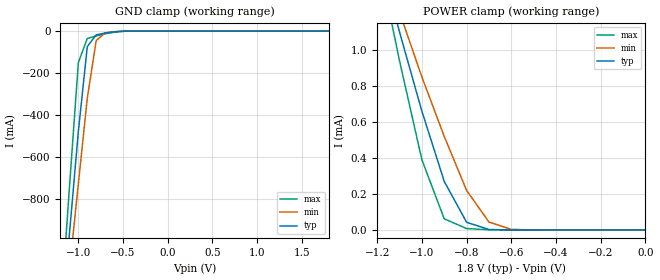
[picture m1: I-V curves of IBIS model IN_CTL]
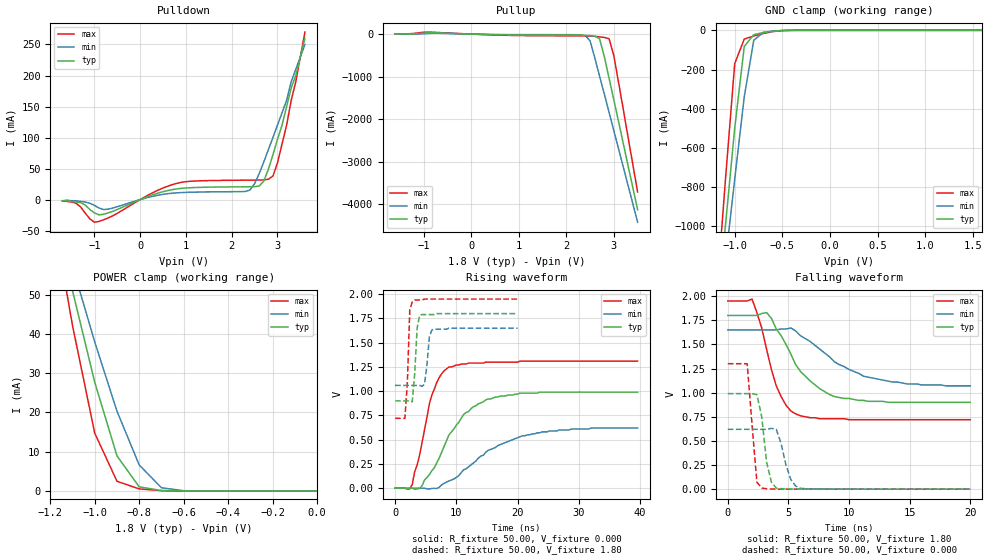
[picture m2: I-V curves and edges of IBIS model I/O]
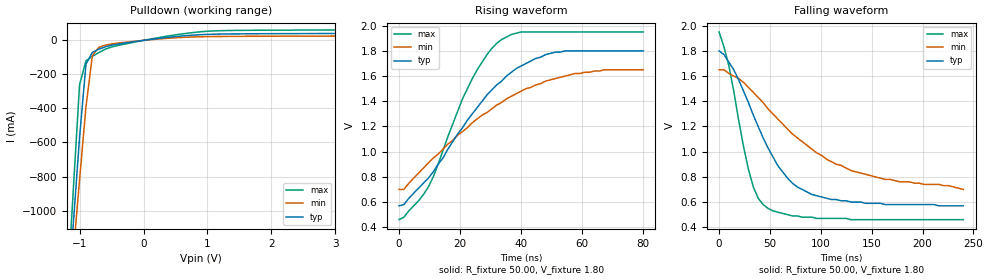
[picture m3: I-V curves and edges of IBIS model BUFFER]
| This IBIS file was created by s2ibis3 version 1.1
| North Carolina State University, ERL, 2006
[IBIS ver] 3.2
[File name] s34ms01g1_b_i_18_r2.ibs
[File Rev] 2.0
|   Rev1.0 Initial release with updated measurement
|   (X16 ONFI F48 98662AE 41087)
|   Rev2.0 Update 0A for 0V
[Date] 07/23/2014
[Source] Spansion IBIS team
|   Email: dl.ibisteam@spansion.com
[Notes]  Generated IBIS models from SPICE simulations.
|   VIO=1.65V - 1.95V, Temperature Range: Industrial (-40oC to +90oC).
[Disclaimer] THE MODEL LIBRARIES ARE PROVIDED AS IS.
[Copyright] (C) COPYRIGHT 2014
| SPANSION LLC
| ALL RIGHTS RESERVED.
|   Component S34MS01G1 X16 ONFI F48 in VBM063 package
[Component]   S34MS01G1
[Manufacturer]   Spansion
[Package]
| variable   typ   min   max
R_pkg   201.77mOhm   180.41mOhm   223.54mOhm
L_pkg   4.10nH   3.29nH   5.20nH
C_pkg   1.27pF   1.10pF   1.60pF
[Pin]   signal_name   model_name   R_pin   L_pin   C_pin
 A1   R   NC
 A2   R   NC
 A9   R   NC
 A10   R   NC
 B1   R   NC
 B9   R   NC
 B10   R   NC
 C3   WP#   BUFFER   223.54m   4.84n   1.60p
 C4   AL   IN_CTL   217.83m   4.92n   1.44p
 C5   VSS   GND
 C6   E#   IN_CTL   189.69m   3.65n   1.15p
 C7   W#   IN_CTL   210.13m   4.21n   1.36p
 C8   RB#   IN_CTL   180.41m   3.32n   1.18p
 D3   VDD   POWER
 D4   R#   IN_CTL   203.67m   4.50n   1.39p
 D5   CL   IN_CTL   192.84m   3.97n   1.24p
 D6   R   NC
 D7   R   NC
 D8   R   NC
 E3   R   NC
 E4   R   NC
 E5   R   NC
 E6   R   NC
 E7   R   NC
 E8   R   NC
 F3   R   NC
 F4   R   NC
 F5   R   NC
 F6   R   NC
 F7   VSS   GND
 F8   R   NC
 G3   R   NC
 G4   VDD   POWER
 G5   R   NC
 G6   I/O13   I/O   191.74m   3.47n   1.12p
 G7   I/O15   I/O   195.49m   3.29n   1.17p
 G8   R   NC
 H3   I/O8   I/O   213.66m   5.20n   1.43p
 H4   I/O0   I/O   209.17m   4.18n   1.39p
 H5   I/O10   I/O   185.98m   4.00n   1.10p
 H6   I/O12   I/O   198.14m   3.38n   1.18p
 H7   I/O14   I/O   191.63m   3.38n   1.16p
 H8   VDD   POWER
 J3   I/O9   I/O   212.31m   5.12n   1.41p
 J4   I/O1   I/O   204.93m   4.77n   1.32p
 J5   I/O11   I/O   196.16m   3.66n   1.14p
 J6   VDD   POWER
 J7   I/O5   I/O   195.51m   3.75n   1.19p
 J8   I/O7   I/O   199.84m   3.81n   1.17p
 K3   VSS   GND
 K4   I/O2   I/O   212.59m   4.62n   1.32p
 K5   I/O3   I/O   198.07m   3.97n   1.15p
 K6   I/O4   I/O   208.64m   4.08n   1.33p
 K7   I/O6   I/O   208.81m   4.22n   1.32p
 K8   VSS   GND
 L1   R   NC
 L2   R   NC
 L9   R   NC
 L10   R   NC
 M1   R   NC
 M2   R   NC
 M9   R   NC
 M10   R   NC
| Models and submodels in the file (3): IN_CTL (Input), I/O (I/O), BUFFER (Open_drain)
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|   Model IN_CTL
[Model]   IN_CTL
Model_type   Input
Vinl =   0.36V
Vinh =   1.44V
C_comp   4.34pF   3.91pF   5.21pF
[Temperature Range]   25.00   90.00   -40.00
[Voltage Range]   1.80V   1.65V   1.95V
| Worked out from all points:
|   GND clamp passes 1 mA (typ) near -0.50 V on its own axis
|   POWER clamp passes 1 mA (typ) near -1.08 V on its own axis
[GND_clamp]
| voltage   I(typ)   I(min)   I(max)
-1.8V     -4.43A     -4.03A     -5.05A
-1.2V     -1.47A     -1.56A     -1.36A
-1.1V     -970mA     -1.14A     -750mA
-1V       -480mA     -730mA     -150mA
-900mV    -73.87mA   -320mA     -35.7mA
-800mV    -17.88mA   -45.12mA   -23.11mA
-700mV    -9.1mA     -8.55mA    -13.23mA
-600mV    -3.69mA    -2.85mA    -5.42mA
-400mV    -110uA     -120uA     -100uA
1.8V      240pA      1.3nA      110pA
[POWER_clamp]
| voltage   I(typ)   I(min)   I(max)
-1.8V     4.52mA     3.92mA     5.46mA
-1.2V     1.57mA     1.59mA     1.54mA
-1.1V     1.1mA      1.21mA     940uA
-1V       660uA      850uA      390uA
-900mV    270uA      520uA      62.17uA
-800mV    42.85uA    220uA      7.81uA
-700mV    2.54uA     43.98uA    890nA
-600mV    180nA      3.36uA     66.87nA
0V        0A         0A         0A
|   Model I/O
[Model]   I/O
Model_type   I/O
Polarity   Inverting
Enable   Active-Low
Vinl  =   0.36V
Vinh  =   1.44V
Vmeas =   0.90V
C_comp   3.48pF   3.13pF   4.18pF
[Temperature Range]   25.00   90.00   -40.00
[Voltage Range]   1.80V   1.65V   1.95V
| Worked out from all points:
|   slope of the pulldown table from 0 to 0.27 V, typ, clamps not added: 35.9 ohm
|   slope of the pullup table from 0 to 0.27 V, typ, clamps not added: 31.6 ohm
|   GND clamp passes 1 mA (typ) near -0.49 V on its own axis
|   POWER clamp passes 1 mA (typ) near -0.80 V on its own axis
|   rising waveform, R_fixture 50.00, V_fixture 0.000: 20-80 % time 5.79ns typ, 8.76ns min, 2.87ns max; typ from 0 V to 0.99 V
|   rising waveform, R_fixture 50.00, V_fixture 1.80: 20-80 % time 512ps typ, 545ps min, 455ps max; typ from 0.9 V to 1.8 V
|   falling waveform, R_fixture 50.00, V_fixture 1.80: 20-80 % time 2.97ns typ, 4.24ns min, 1.66ns max; typ from 1.8 V to 0.9 V
|   falling waveform, R_fixture 50.00, V_fixture 0.000: 20-80 % time 630ps typ, 805ps min, 510ps max; typ from 0.99 V to 0 V
[Pulldown]
| voltage   I(typ)   I(min)   I(max)
-1.7V     -2mA       -2mA       -2mA
-1.4V     -4mA       -2mA       -6mA
-1V       -21.5mA    -9.4mA     -36.5mA
-700mV    -21.55mA   -15.49mA   -29.61mA
800mV     17.17mA    10.84mA    26.12mA
2.3V      20.58mA    13.03mA    31.25mA
2.5V      20.78mA    25.63mA    31.37mA
2.7V      29.72mA    60.45mA    31.69mA
2.9V      71.92mA    100mA      37.76mA
3.2V      150mA      160mA      120mA
3.3V      180mA      190mA      160mA
3.6V      260mA      250mA      270mA
[Pullup]
| voltage   I(typ)   I(min)   I(max)
-1.6V     2.6mA      1.9mA      3.3mA
-900mV    30.55mA    14.19mA    46.85mA
700mV     -18.21mA   -11.31mA   -27.49mA
2.1V      -24.45mA   -14.19mA   -41.16mA
2.4V      -29.59mA   -34.69mA   -42.55mA
2.5V      -36.59mA   -160mA     -45.69mA
2.6V      -47.63mA   -560mA     -53.7mA
2.7V      -110mA     -990mA     -65.37mA
2.8V      -530mA     -1.41A     -79.35mA
2.9V      -1.04A     -1.84A     -110mA
3V        -1.55A     -2.27A     -510mA
3.5V      -4.13A     -4.42A     -3.71A
[GND_clamp]
| voltage   I(typ)   I(min)   I(max)
-1.6V     -3.59A     -3.33A     -3.99A
-1.2V     -1.52A     -1.61A     -1.42A
-1.1V     -1.01A     -1.19A     -780mA
-1V       -500mA     -760mA     -170mA
-900mV    -82.68mA   -340mA     -44.8mA
-800mV    -22.28mA   -50.64mA   -28.91mA
-700mV    -11.42mA   -10.58mA   -16.3mA
-600mV    -4.6mA     -3.62mA    -6.52mA
-400mV    -130uA     -150uA     -120uA
1.6V      290pA      1.71nA     140pA
[POWER_clamp]
| voltage   I(typ)   I(min)   I(max)
-1.8V     240mA      210mA      290mA
-1.2V     76.17mA    77.46mA    74.6mA
-1.1V     51.04mA    57.29mA    42.14mA
-1V       27.7mA     37.97mA    14.73mA
-900mV    8.94mA     20.33mA    2.46mA
-800mV    1.03mA     6.62mA     520uA
-700mV    97.74uA    810uA      68.2uA
-600mV    10.52uA    59.01uA    5.35uA
0V        0A         0A         0A
[Ramp]
| variable   typ   min   max
dV/dt_r   0.58/5.46n   0.31/6.36n   0.78/2.81n
dV/dt_f   0.54/2.91n   0.35/4.33n   0.74/1.55n
R_load = 50.00
[Rising Waveform]
R_fixture = 50.00
V_fixture = 0.000
V_fixture_min = 0.000
V_fixture_max = 0.000
| time   V(typ)   V(min)   V(max)
0s        0V         0V         0V
2.8ns     -26uV      220nV      37.73mV
4ns       -2.35mV    79.58uV    340mV
6ns       180mV      -2.61mV    960mV
7.2ns     310mV      8.53mV     1.14V
8.8ns     550mV      74.68mV    1.25V
11.2ns    760mV      190mV      1.28V
16.4ns    940mV      420mV      1.3V
24ns      990mV      580mV      1.31V
39.6ns    990mV      620mV      1.31V
[Rising Waveform]
R_fixture = 50.00
V_fixture = 1.80
V_fixture_min = 1.65
V_fixture_max = 1.95
| time   V(typ)   V(min)   V(max)
0s        900mV      1.06V      720mV
1.6ns     900mV      1.06V      720mV
2ns       900mV      1.06V      1.08V
2.4ns     900mV      1.06V      1.84V
2.8ns     890mV      1.06V      1.92V
3.6ns     1.65V      1.06V      1.94V
4ns       1.78V      1.06V      1.94V
4.8ns     1.79V      1.07V      1.95V
6ns       1.79V      1.63V      1.95V
20ns      1.8V       1.65V      1.95V
[Falling Waveform]
R_fixture = 50.00
V_fixture = 1.80
V_fixture_min = 1.65
V_fixture_max = 1.95
| time   V(typ)   V(min)   V(max)
0s        1.8V       1.65V      1.95V
2ns       1.8V       1.65V      1.97V
2.8ns     1.82V      1.65V      1.67V
3.2ns     1.83V      1.65V      1.45V
4ns       1.66V      1.65V      1.07V
4.8ns     1.5V       1.66V      870mV
5.6ns     1.29V      1.64V      780mV
8.4ns     980mV      1.37V      730mV
11.2ns    920mV      1.17V      720mV
20ns      900mV      1.07V      720mV
[Falling Waveform]
R_fixture = 50.00
V_fixture = 0.000
V_fixture_min = 0.000
V_fixture_max = 0.000
| time   V(typ)   V(min)   V(max)
0s        990mV      620mV      1.3V
1.6ns     990mV      620mV      1.3V
2.4ns     980mV      620mV      72.85mV
2.8ns     750mV      620mV      12.43mV
3.2ns     280mV      620mV      3.88mV
3.6ns     71.09mV    630mV      1.96mV
4ns       10.62mV    620mV      1.11mV
5.2ns     1.94mV     99.79mV    380uV
6ns       760uV      8.29mV     190uV
20ns      35.13uV    13.85uV    10.73uV
|   Model BUFFER
[Model]   BUFFER
Model_type   Open_drain
Polarity   Non-Inverting
Enable   Active-Low
Vmeas =   0.9000V
Rref =   2.0000k
Vref =   1.8000V
C_comp   3.92pF   3.53pF   4.70pF
[Temperature Range]   25.00   90.00   -40.00
[Voltage Range]   1.80V   1.65V   1.95V
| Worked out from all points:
|   slope of the pulldown table from 0 to 0.27 V, typ, clamps not added: 20.7 ohm
|   rising waveform, R_fixture 50.00, V_fixture 1.80: 20-80 % time 22.8ns typ, 29.6ns min, 15.3ns max; typ from 0.57 V to 1.8 V
|   falling waveform, R_fixture 50.00, V_fixture 1.80: 20-80 % time 44.7ns typ, 85.2ns min, 22ns max; typ from 1.8 V to 0.57 V
[Pulldown]
| voltage   I(typ)   I(min)   I(max)
-1.7V     -4.29A     -3.92A     -4.86A
-1.2V     -1.62A     -1.7A      -1.54A
-1.1V     -1.09A     -1.26A     -890mA
-1V       -570mA     -820mA     -260mA
-900mV    -140mA     -390mA     -120mA
-800mV    -70.59mA   -90.34mA   -94.24mA
-700mV    -51.91mA   -41.16mA   -71.52mA
-400mV    -21.65mA   -15.79mA   -29.77mA
300mV     14.37mA    9.95mA     20.49mA
900mV     33.57mA    21.29mA    50.74mA
1.5V      38.33mA    23.73mA    58.75mA
3.6V      40.97mA    25.68mA    61.9mA
[Ramp]
| variable   typ   min   max
dV/dt_r   0.36/11.11n   0.26/11.19n   0.55/9.56n
dV/dt_f   0.15/11.48n   50.40m/10.06n   0.44/11.38n
R_load = 50.00
[Rising Waveform]
R_fixture = 50.00
V_fixture = 1.80
V_fixture_min = 1.65
V_fixture_max = 1.95
| time   V(typ)   V(min)   V(max)
0s        570mV      700mV      460mV
1.6ns     580mV      700mV      480mV
9.6ns     790mV      910mV      720mV
20.8ns    1.19V      1.16V      1.42V
24ns      1.3V       1.23V      1.58V
28.8ns    1.45V      1.31V      1.77V
33.6ns    1.56V      1.39V      1.89V
40ns      1.68V      1.48V      1.95V
51.2ns    1.79V      1.58V      1.95V
80ns      1.8V       1.65V      1.95V
[Falling Waveform]
R_fixture = 50.00
V_fixture = 1.80
V_fixture_min = 1.65
V_fixture_max = 1.95
| time   V(typ)   V(min)   V(max)
0s        1.8V       1.65V      1.95V
9.6ns     1.71V      1.62V      1.68V
28.8ns    1.39V      1.51V      860mV
33.6ns    1.29V      1.47V      720mV
38.4ns    1.2V       1.43V      630mV
48ns      1.03V      1.34V      550mV
67.2ns    790mV      1.18V      500mV
91.2ns    660mV      1.02V      480mV
129.6ns   600mV      850mV      460mV
240ns     570mV      700mV      460mV
